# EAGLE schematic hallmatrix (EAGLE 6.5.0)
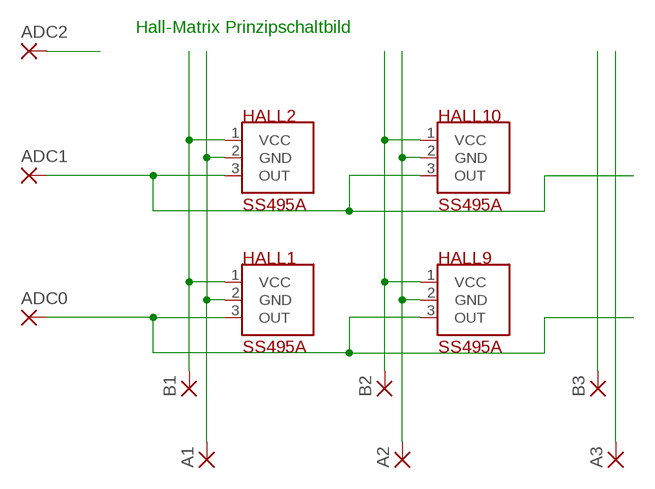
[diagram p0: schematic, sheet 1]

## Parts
A1  WIREPAD2,15/1,0  [2,15/1,0]
A2  WIREPAD2,15/1,0  [2,15/1,0]
A3  WIREPAD2,15/1,0  [2,15/1,0]
ADC0  WIREPAD2,15/1,0  [2,15/1,0]
ADC1  WIREPAD2,15/1,0  [2,15/1,0]
ADC2  WIREPAD2,15/1,0  [2,15/1,0]
B1  WIREPAD2,15/1,0  [2,15/1,0]
B2  WIREPAD2,15/1,0  [2,15/1,0]
B3  WIREPAD2,15/1,0  [2,15/1,0]
HALL1  SS495A  [SS495A]
HALL2  SS495A  [SS495A]
HALL9  SS495A  [SS495A]
HALL10  SS495A  [SS495A]

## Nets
N$1: ADC0.1(P) HALL1.3(OUT) HALL9.3(OUT)
N$2 [dick]: A1.1(P) HALL1.2(GND) HALL2.2(GND)
N$3 [dick]: A2.1(P) HALL9.2(GND) HALL10.2(GND)
N$4 [dick]: B2.1(P) HALL9.1(VCC) HALL10.1(VCC)
N$5 [dick]: B1.1(P) HALL1.1(VCC) HALL2.1(VCC)
N$6: ADC1.1(P) HALL2.3(OUT) HALL10.3(OUT)
N$7: ADC2.1(P)
N$8: B3.1(P)
N$9: A3.1(P)

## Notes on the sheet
- Hall-Matrix Prinzipschaltbild

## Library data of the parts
A1-A3 ADC0 ADC1 ADC2 B1-B3 = wirepad:WIREPAD: Wire PAD connect wire on PCB
HALL1 HALL2 HALL9 HALL10 = hallsensor:SS495A

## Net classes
1 dick: width 0.508 mm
